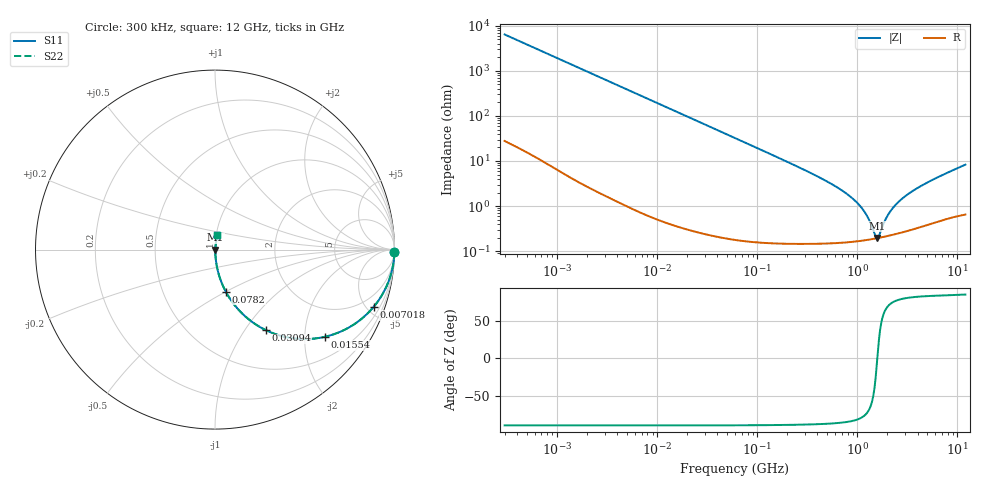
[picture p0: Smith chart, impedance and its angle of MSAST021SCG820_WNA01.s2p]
! MSAST021SCG820_WNA01  S-PARAMETER MODEL  ( Standard Model )
! Model Generated by TAIYO YUDEN Corporation (http://www.ty-top.com)
! Version 1.0
! TAIYO YUDEN Control No. 241126
! Copyright(c) 2024 TAIYO YUDEN CO.,LTD. All Rights Reserved.
! Product Description (link to TY-COMPAS)
! https://ds.yuden.co.jp/TYCOMPAS/or/detail?pn=MSAST021SCG820GWNA01&u=M
! Products Name : Multilayer Ceramic Capacitors
! Characteristics :
!  Capacitance : 82 [pF] , Rated Voltage : 25 [V] , TCC : CG / C0G
!  Case Size : 0.25 x 0.125 / 0.0098 x 0.0049 [mm/inch] , Thickness : 0.125 / 0.0049 [mm/inch]
!  (Conditions: Temperature = 25 [degC] , DC Bias Voltage = 0 [V])
! External Node Assignments :
!  1  o---| |---o  2
! GND o---------o GND
! Frequency Range : 0.3MHz  -  12000MHz  [ 401 STEP ]
# MHZ S RI R 50
! Freq[MHz].  S11 Real  S11 Imag  S21 Real  S21 Imag  S12 Real  S12 Imag  S22 Real  S22 Imag
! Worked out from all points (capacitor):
!   401 points, 300 kHz to 12 GHz, reference 50 ohm
!   read as one part in series: C = 82.3 pF near 316.3 kHz
!   lowest |Z| = 196 mohm at 1.561 GHz (marker M1)
!   series resonance near 1.582 GHz, so ESL is about 120 pH
!   S11 on the Smith chart (normalised r, x): 300 kHz: open; 7.018 MHz: 1.01, -5.54; 15.54 MHz: 1.01, -2.51; 30.94 MHz: 1.00, -1.26; 78.2 MHz: 1.00, -0.50; 12 GHz: 1.01, +0.17
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0.3  0.9997 -0.0155  0.000308 0.0155  0.000308 0.0155  0.9997 -0.0155
1.769972  0.9915 -0.0904  0.0085 0.0904  0.0085 0.0904  0.9915 -0.0904
4.023703  0.9584 -0.1983  0.0416 0.1983  0.0416 0.1983  0.9584 -0.1983
7.018335  0.8842 -0.3188  0.1158 0.3188  0.1158 0.3188  0.8842 -0.3188
10.44266  0.7758 -0.4158  0.2242 0.4158  0.2242 0.4158  0.7758 -0.4158
15.53777  0.6105 -0.4862  0.3895 0.4862  0.3895 0.4862  0.6105 -0.4862
30.94016  0.2845 -0.4493  0.7155 0.4493  0.7155 0.4493  0.2845 -0.4493
60  0.0965 -0.2926  0.9035 0.2926  0.9035 0.2926  0.0965 -0.2926
78.19928  0.0596 -0.2335  0.9404 0.2335  0.9404 0.2335  0.0596 -0.2335
155.7172  0.0166 -0.1218  0.9834 0.1218  0.9834 0.1218  0.0166 -0.1218
353.9943  0.00416 -0.052  0.9958 0.052  0.9958 0.052  0.00416 -0.052
651.0506  0.00213 -0.0247  0.9979 0.0247  0.9979 0.0247  0.00213 -0.0247
968.706  0.00179 -0.0125  0.9982 0.0125  0.9982 0.0125  0.00179 -0.0125
1229.528  0.0018 -0.0062  0.9982 0.0062  0.9982 0.0062  0.0018 -0.0062
1480.043  0.00189 -0.00162  0.9981 0.00162  0.9981 0.00162  0.00189 -0.00162
1560.575  0.00193 -0.000334  0.9981 0.000334  0.9981 0.000334  0.00193 -0.000334
1645.489  0.00197 0.000945  0.998 -0.000945  0.998 -0.000945  0.00197 0.000945
1878.541  0.00211 0.00415  0.9979 -0.00415  0.9979 -0.00415  0.00211 0.00415
2088.533  0.00225 0.00674  0.9977 -0.00674  0.9977 -0.00674  0.00225 0.00674
2650.866  0.00268 0.0128  0.9973 -0.0128  0.9973 -0.0128  0.00268 0.0128
3642.919  0.00354 0.0219  0.9965 -0.0219  0.9965 -0.0219  0.00354 0.0219
12000  0.0132 0.0814  0.9868 -0.0814  0.9868 -0.0814  0.0132 0.0814
